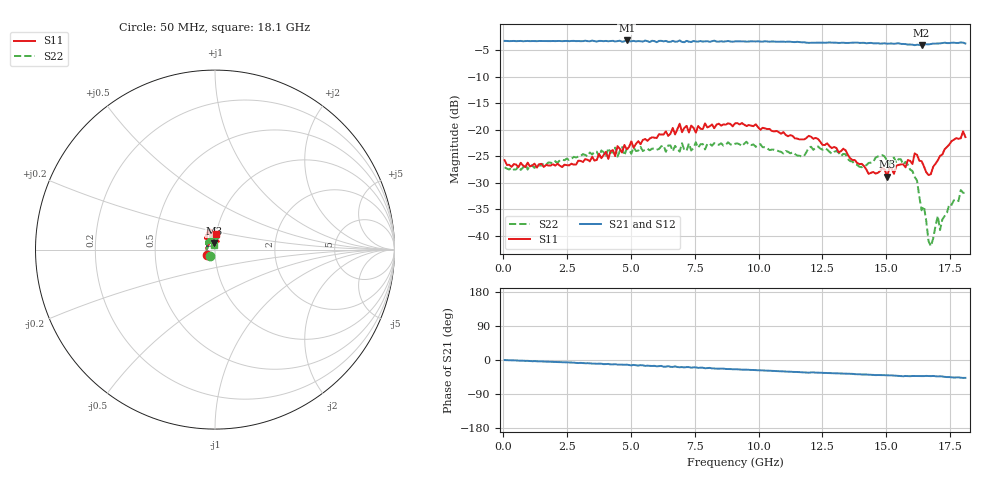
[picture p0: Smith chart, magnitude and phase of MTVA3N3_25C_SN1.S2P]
! Network Analyzer HP8720D.06.14 Serial No. US36140669
! 27 Jun 2005  08:27:20
! Frequency  S11  S21  S12  S22
# HZ  S  DB R 50
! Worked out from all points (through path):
!   201 points, 50 MHz to 18.1 GHz, reference 50 ohm
!   highest |S21| = -3.11 dB at 4.833 GHz (marker M1); lowest = -4.0 dB at 16.39 GHz (marker M2)
!   group delay of S21, straight-line fit = 7.35 ps
!   lowest |S11| = -28.9 dB at 15.03 GHz (marker M3), VSWR 1.07, Z = 49.3 + j3.51 ohm
!   |S11| at or under -10 dB: start of sweep to end of sweep
!   |S22| runs from -42.0 to -22.2 dB; largest |S21 - S12| = 0.02
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5e7  -25.73 -143.9  -3.19 -0.2  -3.21 0.2  -27.06 -124.8
3.1185e9  -26.07 133.1  -3.24 -8.2  -3.25 -8.3  -24.60 146.1
4.83325e9  -23.69 117.4  -3.11 -12.3  -3.15 -13.2  -23.60 125.6
6.09675e9  -20.84 105.3  -3.19 -16.2  -3.16 -16.1  -23.61 112.4
6.909e9  -18.84 105.0  -3.11 -19.1  -3.25 -18.5  -24.11 98.5
9.075e9  -18.77 106.4  -3.29 -24.4  -3.27 -24.4  -22.64 77.6
1.169225e10  -21.80 129.7  -3.47 -32.7  -3.47 -32.5  -25.06 97.3
1.21435e10  -21.69 128.4  -3.56 -32.6  -3.53 -32.8  -23.77 103.0
1.403875e10  -26.43 115.6  -3.57 -38.2  -3.57 -38.4  -27.06 121.2
1.50315e10  -28.88 98.7  -3.72 -40.2  -3.70 -40.8  -25.88 121.1
1.512175e10  -27.21 94.3  -3.69 -40.8  -3.63 -40.4  -26.62 118.0
1.530225e10  -28.32 93.3  -3.76 -41.0  -3.64 -41.8  -25.21 125.5
1.602425e10  -26.45 82.9  -3.91 -42.2  -3.98 -43.5  -27.77 85.4
1.620475e10  -24.72 80.5  -3.92 -42.7  -3.97 -42.3  -29.56 70.5
1.638525e10  -25.92 64.3  -4.03 -42.4  -3.89 -42.2  -35.20 66.5
1.64755e10  -26.89 68.6  -3.92 -42.5  -4.06 -41.6  -34.45 71.6
1.6656e10  -28.53 82.3  -3.86 -42.3  -3.77 -41.7  -41.00 93.7
1.674625e10  -28.38 87.1  -3.78 -42.5  -3.87 -42.7  -41.98 110.8
1.7017e10  -25.78 96.2  -3.69 -43.3  -3.77 -44.0  -36.27 135.5
1.710725e10  -24.92 97.2  -3.67 -43.0  -3.63 -43.3  -38.95 120.6
1.746825e10  -22.78 91.3  -3.61 -45.1  -3.65 -44.8  -34.06 111.2
1.81e10  -21.36 85.2  -3.69 -47.1  -3.69 -48.0  -31.93 98.0
